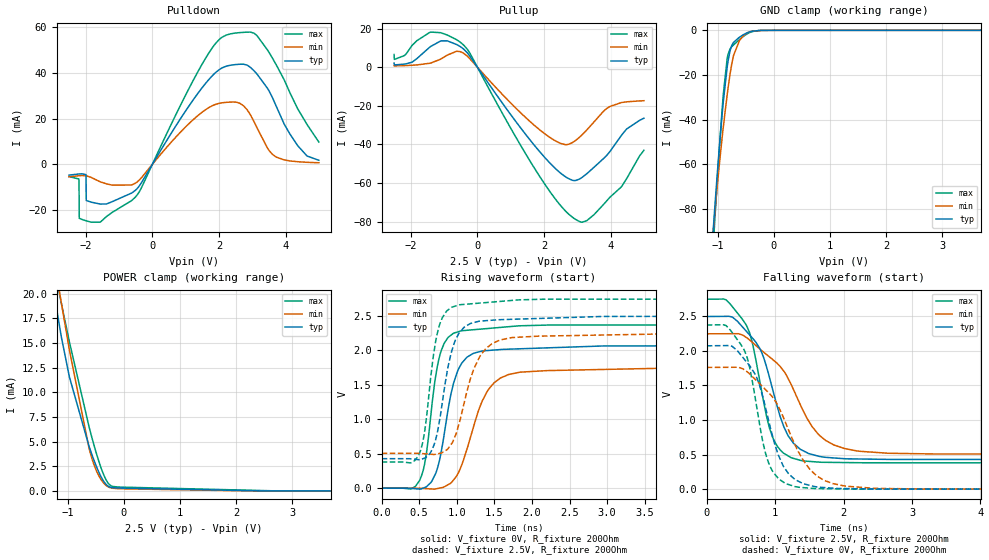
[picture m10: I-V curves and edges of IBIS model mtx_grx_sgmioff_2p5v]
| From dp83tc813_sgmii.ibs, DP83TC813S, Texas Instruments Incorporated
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| mtx_grx_sgmioff_2p5v
[Model]   mtx_grx_sgmioff_2p5v
Model_type   I/O
Polarity   Non-Inverting
Enable   Active-Low
Vinl = 0.7
Vinh = 1.7
Vmeas = 1.25
Vref = 1.25
Cref = 2pF
Rref = 100000
|   typ   min   max
C_comp   3.94pF   4.17pF   3.64pF
[Voltage Range]   2.5   2.25   2.75
[Temperature Range]   27   150   -40
[Pullup Reference]   2.5   2.25   2.75
[Pulldown Reference]   0   -0   -0
[Power Clamp Reference]   2.5   2.25   2.75
[GND Clamp Reference]   0   0   0
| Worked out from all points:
|   slope of the pulldown table from 0 to 0.375 V, typ, clamps not added: 41.3 ohm
|   slope of the pullup table from 0 to 0.375 V, typ, clamps not added: 39.8 ohm
|   GND clamp passes 1 mA (typ) near -0.47 V on its own axis
|   POWER clamp passes 1 mA (typ) near -0.36 V on its own axis
|   falling waveform, V_fixture 2.5V, R_fixture 200Ohm: 20-80 % time 411ps typ, 647ps min, 305ps max; typ from 2.49 V to 0.427 V
|   rising waveform, V_fixture 0V, R_fixture 200Ohm: 20-80 % time 225ps typ, 336ps min, 176ps max; typ from 0 V to 2.07 V
|   rising waveform, V_fixture 2.5V, R_fixture 200Ohm: 20-80 % time 211ps typ, 290ps min, 170ps max; typ from 0.427 V to 2.49 V
|   falling waveform, V_fixture 0V, R_fixture 200Ohm: 20-80 % time 373ps typ, 567ps min, 281ps max; typ from 2.07 V to 0 V
[Pulldown]
|   Voltage   I(typ)   I(min)   I(max)
-2.5V     -4.672mA   -5.389mA   -5.307mA
-2.208V   -4.173mA   -4.935mA   -6.345mA
-2.2V     -4.164mA   -4.928mA   -6.817mA
-2.192V   -4.156mA   -4.921mA   -23.54mA
-2.118V   -4.109mA   -4.872mA   -23.98mA
-1.99V    -4.622mA   -4.94mA    -24.62mA
-1.982V   -15.77mA   -4.953mA   -24.65mA
-617.5mV  -12.48mA   -8.98mA    -15.76mA
1.587V    35.18mA    23.8mA     46.1mA
2.428V    43.51mA    27.27mA    57.25mA
3.147V    39.41mA    15.86mA    56.18mA
5V        1.822mA    727.1uA    9.773mA
[GND Clamp]
|   Voltage   I(typ)   I(min)   I(max)
-2.5V     -652.2mA   -569.8mA   -733.6mA
-1.105V   -97.03mA   -96.32mA   -105.6mA
-1.045V   -75.84mA   -78.96mA   -80.87mA
-925mV    -37.74mA   -48.18mA   -35.57mA
-902.5mV  -31.69mA   -43.06mA   -28.4mA
-835mV    -16.54mA   -28.92mA   -12.69mA
-782.5mV  -9.053mA   -19.51mA   -8.294mA
-722.5mV  -5.45mA    -11.39mA   -6.566mA
-617.5mV  -3.11mA    -4.678mA   -4.182mA
-482.5mV  -1.159mA   -1.256mA   -1.648mA
-197.5mV  -28.29uA   -44.8uA    -30.5uA
5V        0A         0A         0A
[Pullup]
|   Voltage   I(typ)   I(min)   I(max)
-2.5V     2.111mA    768.5uA    6.54mA
-2.2V     1.575mA    804.7uA    5.936mA
-1.96V    2.572mA    997.9uA    11.28mA
-1.39V    10.84mA    2.186mA    18.18mA
-902.5mV  13.62mA    6.256mA    16.65mA
-467.5mV  10.11mA    7.704mA    12.3mA
2.083V    -47.91mA   -35.26mA   -62.11mA
2.638V    -56.7mA    -40.12mA   -74.4mA
3.065V    -57.97mA   -36.33mA   -79.98mA
3.973V    -43.87mA   -20.44mA   -67.55mA
4.482V    -32.02mA   -17.96mA   -57.73mA
5V        -26.43mA   -17.39mA   -43.06mA
[POWER Clamp]
|   Voltage   I(typ)   I(min)   I(max)
-2.5V     127.6mA    94.09mA    171.5mA
-1.232V   19.61mA    23.09mA    22.45mA
-1.113V   15.56mA    19mA       18.96mA
-970mV    11.54mA    14.28mA    15.09mA
-617.5mV  4.476mA    4.246mA    6.44mA
-550mV    3.38mA     2.956mA    5.003mA
-460mV    2.088mA    1.696mA    3.259mA
-355mV    942.8uA    770.4uA    1.589mA
-272.5mV  461.3uA    397.2uA    740.3uA
-197.5mV  326.8uA    269.2uA    451.3uA
-25mV     285.4uA    216.3uA    382.5uA
5V        0A         0A         0A
[Ramp]
R_load = 200
|   typ   min   max
dV/dt_r   1.24075/2.23768e-10   1.05341/3.35527e-10   1.42105/1.75669e-10
dV/dt_f   1.23795/4.0658e-10   1.04174/6.40999e-10   1.41625/3.0318e-10
[Falling Waveform]
V_fixture = 2.5V
V_fixture_min = 2.25V
V_fixture_max = 2.75V
R_fixture = 200Ohm
C_fixture = 0F
|   Time   V(typ)   V(min)   V(max)
0s        2.491V     2.241V     2.74V
340.8ps   2.491V     2.242V     2.675V
584.5ps   2.273V     2.185V     2.355V
718.6ps   2.119V     2.073V     1.865V
966ps     1.431V     1.869V     742.6mV
1.127ns   901.2mV    1.703V     517mV
1.375ns   572mV      1.205V     414.4mV
1.857ns   450.5mV    638.2mV    385.9mV
2.652ns   429.6mV    518.1mV    380.5mV
12ns      427.3mV    504.7mV    379.4mV
[Rising Waveform]
V_fixture = 0V
V_fixture_min = 0V
V_fixture_max = 0V
R_fixture = 200Ohm
C_fixture = 0F
|   Time   V(typ)   V(min)   V(max)
0s        529.8nV    17.63uV    219.4nV
502.6ps   -13.26mV   -277.1uV   107.1mV
589.2ps   16.36mV    -6.385mV   457.3mV
667.5ps   100.1mV    -11.91mV   1.186V
790.7ps   517.9mV    5.285mV    1.986V
923.5ps   1.37V      77.21mV    2.218V
1.06ns    1.799V     320.2mV    2.28V
1.405ns   1.994V     1.403V     2.313V
1.848ns   2.02V      1.681V     2.353V
12ns      2.068V     1.756V     2.368V
[Rising Waveform]
V_fixture = 2.5V
V_fixture_min = 2.25V
V_fixture_max = 2.75V
R_fixture = 200Ohm
C_fixture = 0F
|   Time   V(typ)   V(min)   V(max)
0s        427.3mV    504.7mV    379.4mV
491.8ps   413.4mV    504.4mV    475.8mV
573.9ps   436.2mV    498.3mV    832.8mV
649.3ps   514.8mV    491.8mV    1.568V
775ps     1.009V     505mV      2.382V
923.5ps   1.953V     633.5mV    2.615V
1.035ns   2.252V     956.7mV    2.657V
1.315ns   2.421V     1.923V     2.683V
1.731ns   2.446V     2.182V     2.72V
12ns      2.491V     2.241V     2.74V
[Falling Waveform]
|Gnd
V_fixture = 0V
V_fixture_min = 0V
V_fixture_max = 0V
R_fixture = 200Ohm
C_fixture = 0F
|   Time   V(typ)   V(min)   V(max)
0s        2.068V     1.756V     2.368V
285.3ps   2.071V     1.758V     2.358V
538ps     1.889V     1.73V      2.024V
638.4ps   1.766V     1.652V     1.705V
908.4ps   977.3mV    1.389V     370.6mV
1.114ns   344.8mV    1.052V     106.7mV
1.292ns   138.2mV    637.3mV    36.6mV
1.712ns   23.72mV    128.6mV    6.998mV
2.455ns   2.964mV    11.79mV    1.35mV
12ns      723.4nV    18.84uV    297.2nV
